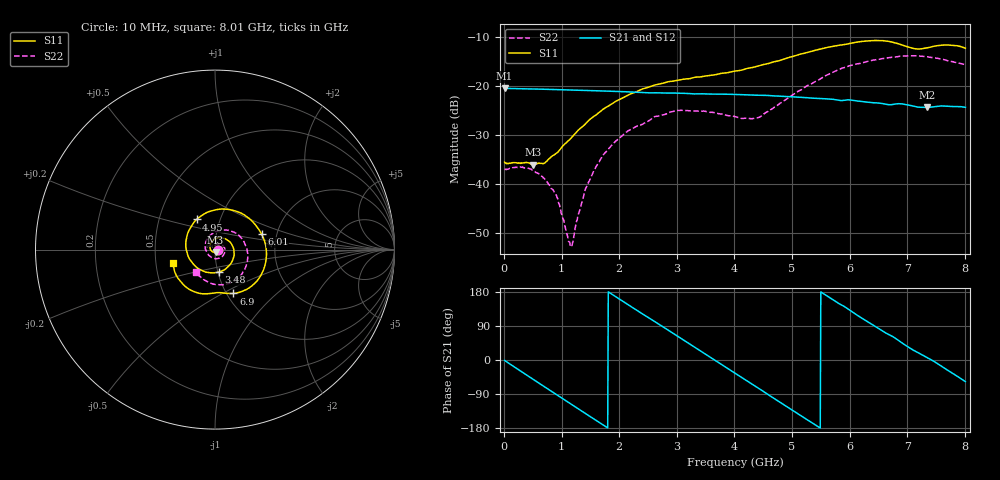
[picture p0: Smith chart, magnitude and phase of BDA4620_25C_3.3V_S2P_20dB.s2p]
!Agilent Technologies,E5071B,MY42404982,A.09.10
!Date: Wed May 06 08:53:02 2026
!Data & Calibration Information:
!Freq	S11:SOLT2(ON)	S21:SOLT2(ON)	S12:SOLT2(ON)	S22:SOLT2(ON)
# Hz S RI R 50
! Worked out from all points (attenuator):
!   801 points, 10 MHz to 8.01 GHz, reference 50 ohm
!   highest |S21| = -20.40 dB at 10 MHz (marker M1); lowest = -24.3 dB at 7.34 GHz (marker M2)
!   lowest |S11| = -36.0 dB at 510 MHz (marker M3), VSWR 1.03, Z = 50.3 - j1.56 ohm
!   |S11| at or under -10 dB: start of sweep to end of sweep
!   |S22| runs from -52.6 to -13.8 dB; largest |S21 - S12| = 0.00041
!   S11 on the Smith chart (normalised r, x): 10 MHz: 1.03, -0.00; 3.48 GHz: 1.01, -0.26; 4.95 GHz: 0.77, +0.27; 6.01 GHz: 1.66, +0.31; 6.9 GHz: 1.07, -0.56; 8.01 GHz: 0.62, -0.10
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1e7  0.0168 -0.0012  0.0954 -0.002  0.0956 -0.00206  0.0141 -0.000489
5.1e8  0.00339 -0.0155  0.0584 -0.0733  0.0585 -0.0735  0.0125 -0.00585
8.9e8  -0.0181 -0.00915  0.00106 -0.0925  0.000978 -0.0927  0.0039 -0.00705
1.15e9  -0.0276 0.00898  -0.039 -0.0829  -0.0391 -0.083  -0.00183 -0.00147
1.19e9  -0.0281 0.0126  -0.0445 -0.0798  -0.0446 -0.0799  -0.00252 -0.000209
1.35e9  -0.0271 0.0271  -0.0643 -0.0643  -0.0643 -0.0644  -0.00422 0.00492
1.56e9  -0.0171 0.0463  -0.082 -0.0372  -0.0822 -0.0371  -0.00369 0.0133
1.83e9  0.0091 0.0629  -0.0889 0.00337  -0.089 0.00338  0.00251 0.0233
2.15e9  0.0518 0.0623  -0.073 0.0485  -0.073 0.0487  0.0176 0.0303
2.68e9  0.105 0.000525  -0.00765 0.0852  -0.00756 0.0853  0.0456 0.0194
3.48e9  0.0211 -0.1249  0.0799 0.0249  0.08 0.0249  0.0402 -0.0385
4.01e9  -0.1044 -0.0972  0.0679 -0.0469  0.0679 -0.047  -0.0118 -0.0477
4.42e9  -0.1615 0.00769  0.0213 -0.0781  0.0212 -0.0782  -0.0464 -0.0128
4.95e9  -0.1026 0.1677  -0.0471 -0.0625  -0.0472 -0.0626  -0.0377 0.0673
5.35e9  0.0358 0.2262  -0.0734 -0.0184  -0.0735 -0.0184  0.0231 0.1043
6.01e9  0.2595 0.087  -0.0469 0.0551  -0.0471 0.0553  0.1508 0.0605
6.35e9  0.2822 -0.0713  -0.00885 0.0678  -0.00889 0.0679  0.1807 -0.0114
6.68e9  0.195 -0.2102  0.0253 0.0597  0.0253 0.0598  0.1722 -0.093
6.9e9  0.1022 -0.2445  0.0459 0.0477  0.0458 0.0478  0.1456 -0.142
7.34e9  -0.0248 -0.2443  0.0604 0.00739  0.0604 0.00747  0.041 -0.1961
7.65e9  -0.1471 -0.2188  0.0582 -0.0235  0.0583 -0.0235  -0.0365 -0.1821
8.01e9  -0.2322 -0.0755  0.0333 -0.051  0.0334 -0.0511  -0.1054 -0.1269
